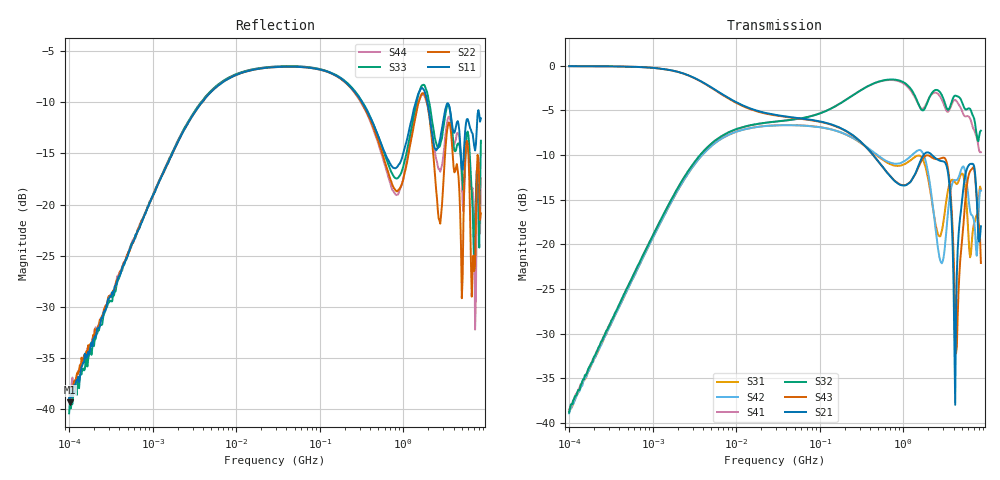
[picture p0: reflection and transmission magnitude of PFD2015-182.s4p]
# MHz S MA R 50
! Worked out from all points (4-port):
!   498 points, 100 kHz to 8.5 GHz, reference 50 ohm
!   strongest paths, dB at 100 kHz, 1.698 MHz, 29.49 MHz, 500.7 MHz, 8.5 GHz:
!     S21: -0.1, -0.5, -5.5, -10.7, -18.0
!     S43: -0.1, -0.5, -5.6, -10.7, -22.1
!     S32: -38.8, -14.9, -6.3, -1.8, -7.3
!     S41: -38.5, -14.9, -6.3, -1.8, -9.7
!     S42: -38.9, -15.2, -6.7, -10.1, -14.0
!     S31: -38.7, -15.1, -6.7, -10.2, -13.8
!   lowest |S11| = -39.4 dB at 102.3 kHz (marker M1), VSWR 1.02, Z = 50.1 + j1.07 ohm
!   |S11| at or under -10 dB: start of sweep to 3.896 MHz; 322.5 MHz to 1.414 GHz (1.091 GHz wide, 126 % of centre); 1.947 GHz to end of sweep
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0.1  0.01127 84.2  0.9929 -0.7  0.01163 -91.5  0.01194 88.4
     0.9929 -0.7  0.01092 85.8  0.01147 87.7  0.01135 -92.9
     0.01163 -91.5  0.01147 87.7  0.009492 73.4  0.9922 -0.6
     0.01194 88.4  0.01135 -92.9  0.9922 -0.6  0.01184 79.9
0.1023101  0.01075 84.1  0.9926 -0.7  0.01176 -92.7  0.01219 87.7
           0.9926 -0.7  0.01156 88.2  0.01207 87.6  0.01187 -92.8
           0.01176 -92.7  0.01207 87.6  0.0108 77.1  0.9927 -0.7
           0.01219 87.7  0.01187 -92.8  0.9927 -0.7  0.01118 81.8
9.200955  0.4245 22.7  0.6374 -19.6  0.4205 -158.2  0.4336 25.2
          0.6374 -19.6  0.4247 22.7  0.4348 25.2  0.4197 -158.4
          0.4205 -158.2  0.4348 25.2  0.428 22.6  0.6323 -19.8
          0.4336 25.2  0.4197 -158.4  0.6323 -19.8  0.4282 22.4
347.4163  0.2999 -78.9  0.3561 -100.8  0.3548 78.4  0.7517 -32.5
          0.3561 -100.8  0.2948 -84.2  0.7517 -32.0  0.3567 74.1
          0.3548 78.4  0.7517 -32.0  0.3031 -79.6  0.3551 -100.7
          0.7517 -32.5  0.3567 74.1  0.3551 -100.7  0.2922 -84.6
1219.999  0.2481 -148.9  0.2236 64.0  0.295 -104.2  0.7293 -170.0
          0.2236 64.0  0.1992 -145.9  0.746 -169.4  0.3102 -108.4
          0.295 -104.2  0.746 -169.4  0.2222 -145.2  0.2244 67.1
          0.7293 -170.0  0.3102 -108.4  0.2244 67.1  0.2068 -145.0
2652.059  0.1939 23.3  0.2959 83.0  0.1119 -97.1  0.6888 9.1
          0.2959 83.0  0.08555 -4.6  0.7228 11.5  0.09057 -61.6
          0.1119 -97.1  0.7228 11.5  0.1907 5.3  0.3 87.8
          0.6888 9.1  0.09057 -61.6  0.3 87.8  0.149 6.3
8500  0.2643 -52.7  0.1263 51.4  0.2043 26.6  0.3279 -29.0
      0.1263 51.4  0.09049 -31.3  0.4325 -35.5  0.1995 2.2
      0.2043 26.6  0.4325 -35.5  0.2053 1.1  0.07873 -5.4
      0.3279 -29.0  0.1995 2.2  0.07873 -5.4  0.1346 2.4
